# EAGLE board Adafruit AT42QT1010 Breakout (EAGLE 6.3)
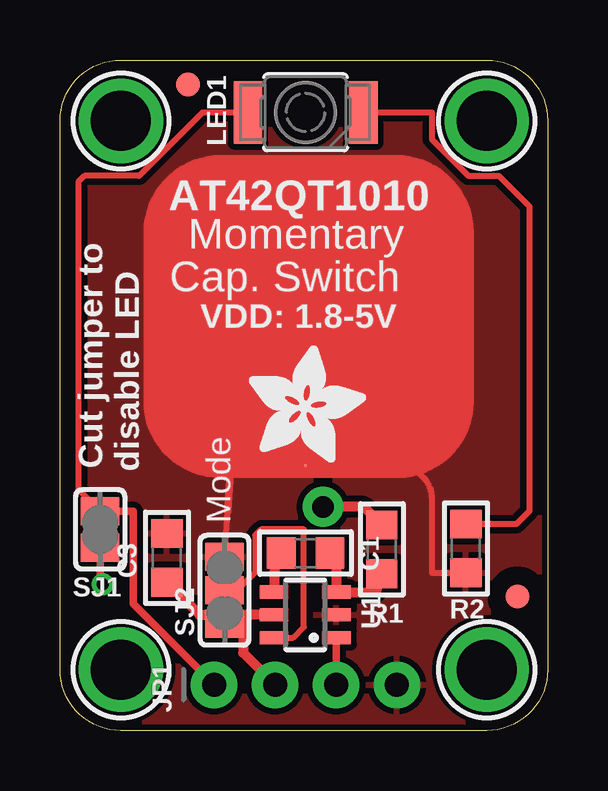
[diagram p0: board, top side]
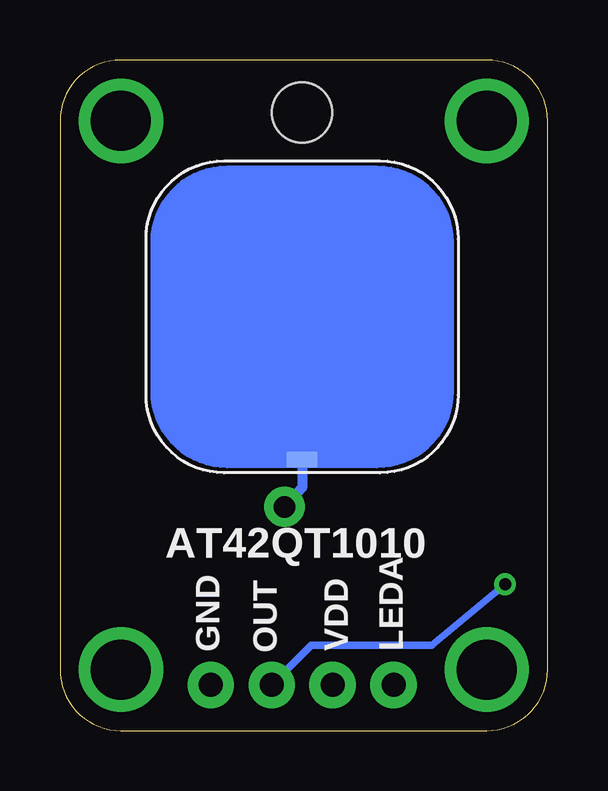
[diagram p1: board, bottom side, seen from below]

Size 20.32 x 27.94 mm. Coordinates in mm from the lower left corner, seen from the top.
Outline: 17.78,0 2.54,0 arc-90 0,2.54 0,25.4 arc-90 2.54,27.94 17.78,27.94 arc-90 20.32,25.4 20.32,2.54 arc-90 17.78,0
Copper layers (1*16): Top 0.035mm / dielectric 1.5mm / Bottom 0.035mm
Design rules "adafruit *": minimum track width 8mil, minimum drill 16mil, track to track 8mil, track to pad 8mil, pad to pad 8mil, via to via 8mil, smd to smd 8mil, copper to edge 10mil, drill to drill 8mil, minimum pad ring 10mil, minimum via ring 8mil, stop-mask expansion 4mil, vias tented up to drill 20mil, thermal gap 10mil
tRestrict: area 4.5,11 to 16,23

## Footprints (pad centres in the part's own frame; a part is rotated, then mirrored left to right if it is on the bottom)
_0805 = smd 1.2 x 1.3: 1 -1.016,0; 2 1.016,0
FIDUCIAL_1MM = smd 1 x 1: 1 0,0
1X04_ROUND_76 = drill 1 pad 1.93: 1 -3.81,0; 2 -1.27,0; 3 1.27,0; 4 3.81,0
PLCC2_REVMOUNT = smd 1.2 x 2.6: A 2.4,0; K -2.4,0 | hole 2.5: 0,0
SOLDERJUMPER_CLOSEDWIRE = smd 1.168 x 1.6: 1 -0.762,0; 2 0.762,0 | smd 0.635 x 0.203: WIRE 0,0
SOLDERJUMPER_2WAY_OPEN_NOPASTE = smd 1.168 x 1.6: 1 -1.397,0; 2 0,0; 3 1.397,0
CAPTOUCH_SIMPLE_12.5MM = smd 1.27 x 0.635: E 0,-5.95 | smd 0.1 x 0.1 bottom: G 0,-6.2
SOT23-6 = smd 0.55 x 1.2: 1 -0.95,-1.3; 2 0,-1.3; 3 0.95,-1.3; 4 0.95,1.3; 5 0,1.3; 6 -0.95,1.3
MOUNTINGHOLE_2.5_PLATED = drill 2.5 pad 3.2: P$1 0,0

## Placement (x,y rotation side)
C1  22nF  [_0805]  10.23,7.4 180 top
C3  0.1µF  [_0805]  4.46,7.2 90 top
FID1  FIDUCIAL""  [FIDUCIAL_1MM]  19.07,5.59 0 top
FID2  FIDUCIAL""  [FIDUCIAL_1MM]  5.33,26.92 0 top
JP1  [1X04_ROUND_76]  10.23,1.91 0 top
LED1  LS T77K-J1L2-1-0-2-R18-Z  [PLCC2_REVMOUNT]  10.23,25.76 180 top
R1  10K  [_0805]  13.41,7.55 90 top
R2  1K  [_0805]  16.91,7.59 270 top
SJ1  LED  [SOLDERJUMPER_CLOSEDWIRE]  1.68,8.38 90 top
SJ2  MODE  [SOLDERJUMPER_2WAY_OPEN_NOPASTE]  6.86,5.84 90 top
SW1  Cap pad  [CAPTOUCH_SIMPLE_12.5MM]  10.23,17.24 0 bottom
U1  AT42QT1010  [SOT23-6]  10.22,4.82 90 top
U$6  MOUNTINGHOLE2.5  [MOUNTINGHOLE_2.5_PLATED]  17.78,2.54 0 top
U$9  MOUNTINGHOLE2.5  [MOUNTINGHOLE_2.5_PLATED]  2.54,2.54 0 top
U$10  MOUNTINGHOLE2.5  [MOUNTINGHOLE_2.5_PLATED]  17.78,25.4 0 top
U$11  MOUNTINGHOLE2.5  [MOUNTINGHOLE_2.5_PLATED]  2.54,25.4 0 top
U$12  [ADAFRUIT_5MM]  7.87,11.18 0 top

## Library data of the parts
C1 C3 FID1 FID2 JP1 LED1 R1 R2 SJ1 SJ2 SW1 U1 U$6 U$9-U$12 = microbuilder

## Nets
CAPPAD: R1.2 SW1.E
GND: C3.2 JP1.4 R2.2 SJ2.3 SW1.G U1.2
LEDA: JP1.1 LED1.A SJ1.2
N$3: C1.2 U1.4
N$4: C1.1 R1.1 U1.3
N$6: LED1.K R2.1
OUT: JP1.3 SJ1.1 U1.1
VDD: C3.1 JP1.2 SJ2.1 SJ2.2 U1.5 U1.6

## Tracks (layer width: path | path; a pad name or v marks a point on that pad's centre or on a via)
CAPPAD  (via drill 0.9 pad 1.68)
  Top 0.406: R1.2 12.65,9.32 v10.96,9.32
  Bottom 0.406: SW1.E 10.23,10.11 v10.96,9.32
GND
  Top 0.254: 14.08,11.03 arc-90 15.49,9.62 15.49,6.6 arc90 15.53,6.57 R2.2 | SJ2.3 6.99,9.15 7,9.15
  Top 0.305: 7,9.15 7.11,11.04
  Top 1.016: SW1.G 7.11,11.04 6.67,11.04 arc-90 3.98,13.73 3.98,20.73 arc-90 6.73,23.48 13.98,23.48 | 13.98,23.48 arc-90 16.73,20.73 16.73,13.73 arc-90 14.08,11.03 10.33,11.03 | 14.03,23.43 arc-90 13.98,23.48
  pour Top (isolate 0.254): 0,0 0,28.7 20.32,28.7 20.32,0
LEDA
  Top 0.254: SJ1.2 0.76,10.06 0.76,22.86 1.02,23.11 3.3,23.11 5.95,25.76 LED1.A
  Top 0.305: JP1.1 3.05,5.28 3.05,9.14 SJ1.2
N$3
  Top 0.406: U1.4 8.96,7 C1.2
N$4
  Top 0.406: C1.1 11.52,7.12 U1.3 13.16,5.77 R1.1
N$6
  Top 0.254: LED1.K 15.49,25.76 15.49,24.64 17.02,23.11 18.29,23.11 19.56,21.84 19.56,9.14 19.02,8.6 R2.1
  Top 0.406: 12.68,25.8 LED1.K
OUT  (via drill 0.5)
  Top 0.305: SJ1.1 1.68,6.45 v1.78,6.1 | U1.1 11.52,1.93 JP1.3
  Bottom 0.305: v1.78,6.1 4.83,3.56 9.85,3.56 JP1.3
VDD
  Top 0.254: 8.86,3.81 U1.6 9.71,3.87 10.16,4.32 10.16,8.38 8.38,8.38 8.13,8.13 8.13,6.6 7.62,6.1 7.11,6.1 SJ2.2 SJ2.1 6.86,5.07
  Top 0.305: 5.82,4.82 6.48,4.82 SJ2.1
  Top 0.406: U1.5 7.73,4.82 | 7.73,4.82 7.63,4.72 7.63,3.23 JP1.2 | C3.1 5.82,4.82 7.73,4.82

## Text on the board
tPlace: AT42QT1010 | Momentary | Cap. Switch | VDD: 1.8-5V | Cut jumper to | disable LED | Mode
bPlace: AT42QT1010 | LEDA | VDD | OUT | GND

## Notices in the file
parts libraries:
microbuilder: This work is placed in the public domain, and may be freely used for commercial and non-commercial work with the following conditions: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
